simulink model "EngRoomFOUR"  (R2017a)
settings: Solver=VariableStepAuto  StartTime=0.0  StopTime=10.0  RelTol=1e-3
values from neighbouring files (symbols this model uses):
  EngDat = engine_pre()    [run_master.m]    (also in engine_pre.m = [MCR1, BSFC1, x)
undefined symbols (not defined in the file or in its folder): num

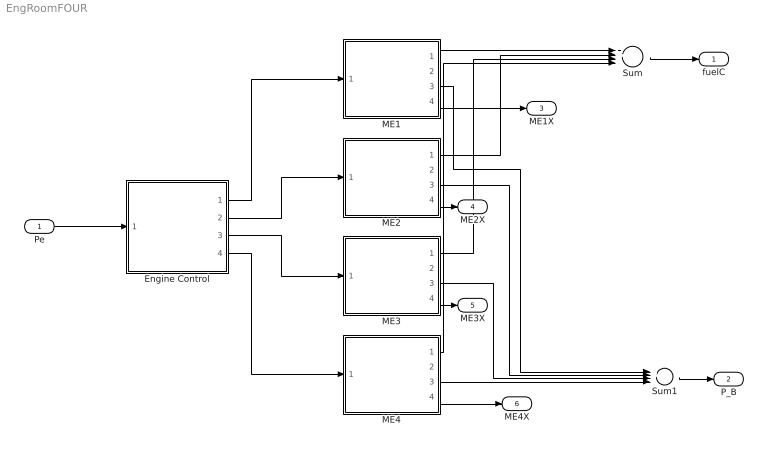
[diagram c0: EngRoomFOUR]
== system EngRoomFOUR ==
  Pe : Inport
  Engine Control : MATLAB Function  TreatAsAtomicUnit=on
  ME1 : MATLAB Function  TreatAsAtomicUnit=on
  ME2 : MATLAB Function  TreatAsAtomicUnit=on
  ME3 : MATLAB Function  TreatAsAtomicUnit=on
  ME4 : MATLAB Function  TreatAsAtomicUnit=on
  Sum : Sum  Inputs=4
  Sum1 : Sum  Inputs=4
  fuelC : Outport
  P_B : Outport  Port=2
  ME1X : Outport  Port=3
  ME2X : Outport  Port=4
  ME3X : Outport  Port=5
  ME4X : Outport  Port=6
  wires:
  Pe/1 -> Engine Control/1(Pe)
  Engine Control/1(P1) -> ME1/1("Pb ")
  Engine Control/2(P2) -> ME2/1("Pb ")
  Engine Control/3(P3) -> ME3/1("Pb ")
  Engine Control/4(P4) -> ME4/1("Pb ")
  Sum/1 -> fuelC/1
  ME1/1(fuel_cons) -> Sum/1
  ME2/1(fuel_cons) -> Sum/2
  ME3/1(fuel_cons) -> Sum/3
  ME4/1(fuel_cons) -> Sum/4
  Sum1/1 -> P_B/1
  ME1/3(Pb) -> Sum1/1
  ME2/3(Pb) -> Sum1/2
  ME3/3(Pb) -> Sum1/3
  ME4/3(Pb) -> Sum1/4
  ME4/4(x) -> ME4X/1
  ME3/4(x) -> ME3X/1
  ME2/4(x) -> ME2X/1
  ME1/4(x) -> ME1X/1

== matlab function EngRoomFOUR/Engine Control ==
function [P1, P2, P3, P4] = fcn(Pe,EngDat)
%take in the total propulsive powering need and Machinery data

%find the optimal settings so that each engine runs close to optimum
%output the load (and rpm) for each engine

%Pe is the required effective power to overcome resistance, the break power
%needed from the engineroom depends on the efficiency of the propulsion
%system, which in turn depends on the configuration of the engines and
%propulsors

% EngDat=([MCR,BSFC,x])

%Read data about the engines from the workspace

%capacity of each engine
PMCR1=EngDat(1,1);
PMCR2=EngDat(2,1);
PMCR3=EngDat(3,1);
PMCR4=EngDat(4,1);

%pre-set to 0
P1=0;
P2=0;
P3=0;
P4=0;
%% Convert Pe into Pb required from the machinery
eta_D = 0.55;
eta_M = 0.95*0.98;
eta_T = eta_D* eta_M;   %Total efficiency
Pb = (Pe/eta_T); %kW

  if Pb<=PMCR4 % If the required load is less than capacity of eng 4
            P1=0; 
            P2=0;
            P3=0;
            P4=Pb;
            return
  elseif Pb<=PMCR3 % If the required load is less than capacity of eng 3
            P1=0; 
            P2=0;
            P3=Pb;
            P4=0;
            return
  elseif Pb<=PMCR2 % If the required load is less than capacity of eng 2
            P1=0;
            P2=Pb;
            P3=0;
            P4=0;
            return
  elseif Pb<=PMCR1
            P1=Pb;
            P2=0;
            P3=0;
            P4=0;
            return
  elseif Pb<=(PMCR4+PMCR3)
            load=Pb/(PMCR4+PMCR3);
            P4=load*PMCR4;
            P3=load*PMCR3;
            return
  elseif Pb<=(PMCR4+PMCR2)
            load=Pb/(PMCR4+PMCR2);
            P4=load*PMCR4;
            P2=load*PMCR2;
            return
  elseif Pb<=(PMCR4+PMCR1)  %4 AND 1
            load=Pb/(PMCR1+PMCR4);
            P1=load*PMCR1;
            P4=load*PMCR4;
            return
  elseif Pb<=(PMCR3+PMCR2)  %3 AND 2
            load=Pb/(PMCR3+PMCR2);
            P3=load*PMCR3;
            P2=load*PMCR2;
            return            
  elseif Pb<=(PMCR3+PMCR1)  %3 AND 1
            load=Pb/(PMCR1+PMCR3);
            P1=load*PMCR1;
            P3=load*PMCR3;
            return 
  elseif Pb<=(PMCR2+PMCR1)  %2 AND 1
            load=Pb/(PMCR1+PMCR2);
            P1=load*PMCR1;
            P2=load*PMCR2;
            return           
  elseif Pb<=(PMCR4+PMCR3+PMCR2)
            load=Pb/(PMCR4+PMCR3+PMCR2);
            P4=load*PMCR4;
            P3=load*PMCR3;
            P2=load*PMCR2;
            return
  elseif Pb<=(PMCR4+PMCR2+PMCR1)
            load=Pb/(PMCR4+PMCR2+OMCR1);
            P4=load*PMCR4;
            P2=load*PMCR2;
            return
  elseif Pb<=(PMCR4+PMCR3+PMCR1)
            load=Pb/(PMCR1+PMCR4+PMCR3);
            P1=load*PMCR1;
            P3=load*PMCR3;
            P4=load*PMCR4;
            return
  elseif Pb<=(PMCR3+PMCR2+PMCR1)
            load=Pb/(PMCR3+PMCR2+PMCR1);
            P3=load*PMCR3;
            P2=load*PMCR2;
            P1=load*PMCR1;
            return
  else 
            load=Pb/(PMCR4+PMCR3+PMCR2+PMCR1);
            P4=load*PMCR4;
            P3=load*PMCR3;
            P2=load*PMCR2;
            P1=load*PMCR1;
  end
  
 
end

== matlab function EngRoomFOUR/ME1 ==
function [fuel_cons,nshaft, Pb, x] = fcn(Pb, num, EngDat)


PMCR=EngDat(1,1);
x = Pb/PMCR; %percentage of maximum
BSFC=EngDat(1,2); %g/kWh
delta_BSFC = 6610.6*x^6 - 20524*x^5 + 23791*x^4 - 11985*x^3 + 1803.2*x^2 + 340.12*x - 36.733;


fuel_cons = (delta_BSFC+BSFC)*Pb/1000; %kg/h

nshaft=neng;


end

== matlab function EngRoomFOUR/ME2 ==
function [fuel_cons,nshaft, Pb, x] = fcn(Pb, num, EngDat)


PMCR=EngDat(2,1);
x = Pb/PMCR; %percentage of maximum
BSFC=EngDat(2,2); %g/kWh
delta_BSFC = 6610.6*x^6 - 20524*x^5 + 23791*x^4 - 11985*x^3 + 1803.2*x^2 + 340.12*x - 36.733;


fuel_cons = (delta_BSFC+BSFC)*Pb/1000; %kg/h

nshaft=neng;


end

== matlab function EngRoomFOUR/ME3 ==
function [fuel_cons,nshaft, Pb, x] = fcn(Pb, num, EngDat)


PMCR=EngDat(3,1);
x = Pb/PMCR; %percentage of maximum
BSFC=EngDat(3,2); %g/kWh
delta_BSFC = 6610.6*x^6 - 20524*x^5 + 23791*x^4 - 11985*x^3 + 1803.2*x^2 + 340.12*x - 36.733;


fuel_cons = (delta_BSFC+BSFC)*Pb/1000; %kg/h

nshaft=neng;


end

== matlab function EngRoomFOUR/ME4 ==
function [fuel_cons,nshaft, Pb, x] = fcn(Pb, num, EngDat)


PMCR=EngDat(4,1);
x = Pb/PMCR; %percentage of maximum
BSFC=EngDat(4,2); %g/kWh
delta_BSFC = 6610.6*x^6 - 20524*x^5 + 23791*x^4 - 11985*x^3 + 1803.2*x^2 + 340.12*x - 36.733;


fuel_cons = (delta_BSFC+BSFC)*Pb/1000; %kg/h

nshaft=neng;


end
